FUNCTION_BLOCK "Main"
VERSION : 0.1
   VAR_TEMP
      compResult : Bool;
   END_VAR


BEGIN
NETWORK
TITLE =
      L INT#1000;
      L INT#500;
      -I;
      <>I;
      = #compResult;
      CALL "__CPROVER_assert"
      (  condition                   := #compResult
      );
      +I;
      L INT#1500;
      ==I;
      = #compResult;
      CALL "__CPROVER_assert"
      (  condition                   := #compResult
      );
      L INT#2;
      *I;
      L INT#3000;
      <=I;
      = #compResult;
      CALL "__CPROVER_assert"
      (  condition                   := #compResult
      );
      L INT#3001;
      <I;
      = #compResult;
      CALL "__CPROVER_assert"
      (  condition                   := #compResult
      );
      L INT#2;
      /I;
      L INT#1500;
      >=I;
      = #compResult;
      CALL "__CPROVER_assert"
      (  condition                   := #compResult
      );
      L INT#1499;
      >I;
      = #compResult;
      CALL "__CPROVER_assert"
      (  condition                   := #compResult
      );
NETWORK
TITLE =
      L DINT#1000;
      L DINT#500;
      -D;
      <>D;
      = #compResult;
      CALL "__CPROVER_assert"
      (  condition                   := #compResult
      );
      +D;
      L DINT#1500;
      ==D;
      = #compResult;
      CALL "__CPROVER_assert"
      (  condition                   := #compResult
      );
      L DINT#2;
      *D;
      L DINT#3000;
      <=D;
      = #compResult;
      CALL "__CPROVER_assert"
      (  condition                   := #compResult
      );
      L DINT#3001;
      <D;
      = #compResult;
      CALL "__CPROVER_assert"
      (  condition                   := #compResult
      );
      L DINT#2;
      /D;
      L DINT#1500;
      >=D;
      = #compResult;
      CALL "__CPROVER_assert"
      (  condition                   := #compResult
      );
      L DINT#1499;
      >D;
      = #compResult;
      CALL "__CPROVER_assert"
      (  condition                   := #compResult
      );
NETWORK
TITLE =
      L 1000.0;
      L 500.0;
      -R;
      <>R;
      = #compResult;
      CALL "__CPROVER_assert"
      (  condition                   := #compResult
      );
      +R;
      L 1500.0;
      ==R;
      = #compResult;
      CALL "__CPROVER_assert"
      (  condition                   := #compResult
      );
      L 2.0;
      *R;
      L 3000.0;
      <=R;
      = #compResult;
      CALL "__CPROVER_assert"
      (  condition                   := #compResult
      );
      L 3001.0;
      <R;
      = #compResult;
      CALL "__CPROVER_assert"
      (  condition                   := #compResult
      );
      L 2.0;
      /R;
      L 1500.0;
      >=R;
      = #compResult;
      CALL "__CPROVER_assert"
      (  condition                   := #compResult
      );
      L 1499.0;
      >R;
      = #compResult;
      CALL "__CPROVER_assert"
      (  condition                   := #compResult
      );
END_FUNCTION_BLOCK

